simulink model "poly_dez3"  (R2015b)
settings: Solver=VariableStepAuto  StartTime=0.0  StopTime=15  RelTol=1e-3
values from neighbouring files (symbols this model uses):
  g = firpolyphase(hdez, M)    [poly_dez_1.m]    (also in poly_dez_2.m; poly_interp_1.m = firpolyphase(hint, L); poly_interp_2.m = firpolyphase(hint, L))
undefined symbols (not defined in the file or in its folder): fir1
libraries: simulink x1

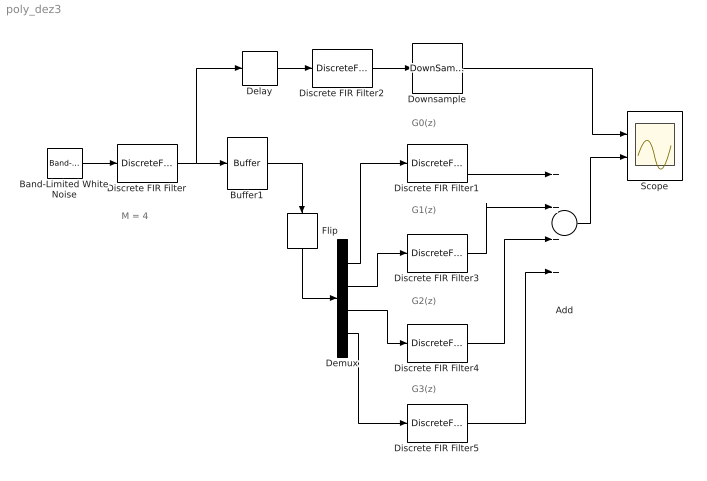
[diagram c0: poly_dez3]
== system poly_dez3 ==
  note: G3(z)
  note: G2(z)
  note: G1(z)
  note: G0(z)
  note: M = 4
  Add : Sum  Inputs=++++
  Band-Limited White Noise : simulink/Sources/Band-Limited White Noise  Cov=[0.1]  Ts=0.1  seed=[23341]
  Buffer1 : Buffer  N=4  TreatMby1Signals=One channel  OutputFrames=off
  Delay : Delay  DelayLength=1
  Demux : Demux
  Discrete FIR Filter : DiscreteFir  Coefficients=fir1(128, 0.2)
  Discrete FIR Filter1 : DiscreteFir  Coefficients=(g(1,:))
  Discrete FIR Filter2 : DiscreteFir  Coefficients=fir1(32,1/4)
  Discrete FIR Filter3 : DiscreteFir  Coefficients=(g(2,:))
  Discrete FIR Filter4 : DiscreteFir  Coefficients=(g(3,:))
  Discrete FIR Filter5 : DiscreteFir  Coefficients=(g(4,:))
  Downsample : DownSample  N=4  RateOptions=Allow multirate processing
  Flip : DSPFlip
  Scope : Scope  NumInputPorts=2
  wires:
  Band-Limited White Noise/1 -> Discrete FIR Filter/1
  Discrete FIR Filter1/1 -> Add/1
  Discrete FIR Filter3/1 -> Add/2
  Discrete FIR Filter4/1 -> Add/3
  Add/1 -> Scope/2
  Discrete FIR Filter5/1 -> Add/4
  Downsample/1 -> Scope/1
  Discrete FIR Filter/1 -> Delay/1, Buffer1/1
  Demux/4 -> Discrete FIR Filter5/1
  Buffer1/1 -> Flip/1
  Demux/1 -> Discrete FIR Filter1/1
  Demux/3 -> Discrete FIR Filter4/1
  Demux/2 -> Discrete FIR Filter3/1
  Flip/1 -> Demux/1
  Discrete FIR Filter2/1 -> Downsample/1
  Delay/1 -> Discrete FIR Filter2/1
